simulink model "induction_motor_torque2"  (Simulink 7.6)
settings: Solver=ode15s  StartTime=0.0  StopTime=20.0  RelTol=1e-3
InitFcn:
  | % valeurs des composants électriques
  | R1=1;
  | R2=1;
  | L1=0.02;
  | L2=0.02;
  | Lm=0.5;
  | n=3;
  | p=1;
  | 
  | % signal d'alimentation des phases du stator
  | Vrms=220/sqrt(2);
  | f=60;
libraries: fl_lib x5, nesl_utility x4, elec_lib x1

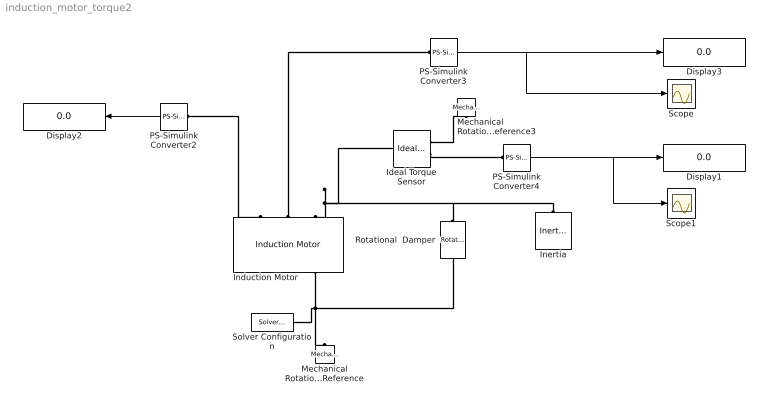
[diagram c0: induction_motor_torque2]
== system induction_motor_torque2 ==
  Display1 : Display
  Display2 : Display
  Display3 : Display
  Ideal Torque Sensor : fl_lib/Mechanical/Mechanical Sensors/Ideal Torque Sensor  DialogController=NetworkEngine.DynNeDlgSource  SystemSampleTime=-1  w_Log=off  t_Log=off  LocalVarNames=|w|t  LocalVarDescs=|w|t  LocalVarLogging=[0 0]
  Induction Motor : elec_lib/Actuators & Drivers/Rotational Actuators/Induction Motor  DialogController=NetworkEngine.DynNeDlgSource  SystemSampleTime=-1  param=2  R1=R1 Ohm  R2=R2 Ohm  L1=L1 H  L2=L2 H  Lm=Lm H  P_rated=825 W  w_mech=3.5e+03 rpm  v_rated=200 V  w_rated=60 Hz  i_rated=2.7 A  paramL=1  i_start=7.5 A  T_max=3.3 N*m  paramR1=1  E=95  pf=0.93  R1m=1 Ohm  V=Vrms V  w=f Hz  p=p  n=n  paramLoad=1  J=0.001 kg*m^2  lam=1e-04 N*m/(rad/s)  speed0=0 rpm  LocalVarLogging=[]
  Inertia : fl_lib/Mechanical/Rotational Elements/Inertia  DialogController=NetworkEngine.DynNeDlgSource  SystemSampleTime=-1  inertia=0.01 kg*m^2  initial_velocity=0 rad/s  t_Log=off  LocalVarNames=|t  LocalVarDescs=|t  LocalVarLogging=0
  Mechanical Rotational Reference : fl_lib/Mechanical/Rotational Elements/Mechanical Rotational Reference  DialogController=NetworkEngine.DynNeDlgSource  SystemSampleTime=-1  t_Log=off  LocalVarNames=|t  LocalVarDescs=|t  LocalVarLogging=0
  Mechanical Rotational Reference3 : fl_lib/Mechanical/Rotational Elements/Mechanical Rotational Reference  DialogController=NetworkEngine.DynNeDlgSource  SystemSampleTime=-1  t_Log=off  LocalVarNames=|t  LocalVarDescs=|t  LocalVarLogging=0
  PS-Simulink Converter2 : nesl_utility/PS-Simulink Converter  DialogController=NetworkEngine.DynNeUtilDlgSource  SystemSampleTime=-1  PhysicalDomain=network_engine_domain  LeftPortType=input  RightPortType=output  SubClassName=ps_output  Unit=rad/s  AffineConversion=off
  PS-Simulink Converter3 : nesl_utility/PS-Simulink Converter  DialogController=NetworkEngine.DynNeUtilDlgSource  SystemSampleTime=-1  PhysicalDomain=network_engine_domain  LeftPortType=input  RightPortType=output  SubClassName=ps_output  Unit=1  AffineConversion=off
  PS-Simulink Converter4 : nesl_utility/PS-Simulink Converter  DialogController=NetworkEngine.DynNeUtilDlgSource  SystemSampleTime=-1  PhysicalDomain=network_engine_domain  LeftPortType=input  RightPortType=output  SubClassName=ps_output  Unit=N*m  AffineConversion=off
  Rotational  Damper : fl_lib/Mechanical/Rotational Elements/Rotational Damper  DialogController=NetworkEngine.DynNeDlgSource  SystemSampleTime=-1  D=0.001 N*m/(rad/s)  t_Log=off  w_Log=off  LocalVarNames=|t|w  LocalVarDescs=|t|w  LocalVarLogging=[0 0]
  Scope : Scope
  Scope1 : Scope
  Solver Configuration : nesl_utility/Solver Configuration  DialogController=NetworkEngine.DynNeUtilDlgSource  SystemSampleTime=-1  PhysicalDomain=network_engine_domain  LeftPortType=input  RightPortType=generic  SubClassName=solver  Accelerate=off  Profile=off  ResidualTolerance=1e-9  MaxNonlinIter=12  MaxModeIter=2  DoFixedCost=off  UseLocalSampling=off  DoDC=off  LinearAlgebra=Sparse  LocalSolverSampleTime=.001  LocalSolverChoice=NE_BACKWARD_EULER_ADVANCER  UseLocalSolver=off
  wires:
  PS-Simulink Converter4/1 -> Display1/1, Scope1/1
  PS-Simulink Converter3/1 -> Display3/1, Scope/1
  PS-Simulink Converter2/1 -> Display2/1
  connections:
  Induction Motor/RConn3 -- Mechanical Rotational Reference/LConn1 -- Solver Configuration/RConn1 -- Rotational  Damper/RConn1
  Induction Motor/LConn3 -- Ideal Torque Sensor/LConn1 -- Rotational  Damper/LConn1 -- Inertia/LConn1
  Ideal Torque Sensor/RConn2 -- PS-Simulink Converter4/LConn1
  Ideal Torque Sensor/RConn1 -- Mechanical Rotational Reference3/LConn1
  Induction Motor/LConn2 -- PS-Simulink Converter3/LConn1
  PS-Simulink Converter2/LConn1 -- Induction Motor/LConn1
